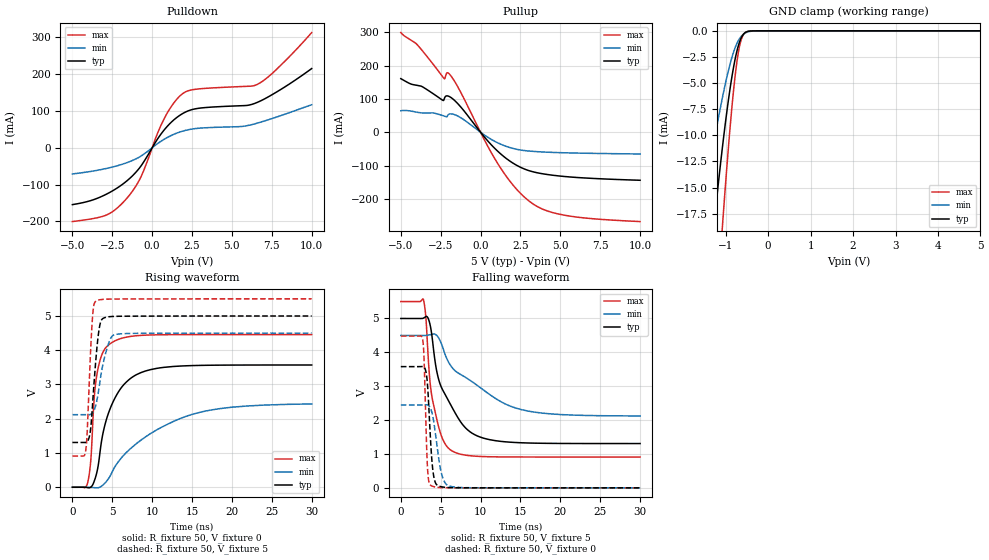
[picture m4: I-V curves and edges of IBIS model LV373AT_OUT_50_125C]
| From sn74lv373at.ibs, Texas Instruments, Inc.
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[Model]   LV373AT_OUT_50_125C
Model_type  3-state
Enable   Active-Low
Vref =   0
Rref =   1000
Cref =   50p
Vmeas =   1.5
| variable   typ   min   max
C_comp   4.53pF   3.43pF   5.27pF
| C_pullup   7.19pF   3.83pF   11.86pF
| C_pulldown   6.90pF   4.00pF   11.55pF
| C_tri-state   4.53pF   3.43pF   5.27pF
[Temperature Range]   40   140   -40
| Ambient temperature   25   125   -40
[Voltage range]   5   4.5   5.5
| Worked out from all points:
|   slope of the pulldown table from 0 to 0.75 V, typ, clamps not added: 15.5 ohm
|   slope of the pullup table from 0 to 0.75 V, typ, clamps not added: 18 ohm
|   GND clamp passes 1 mA (typ) near -0.67 V on its own axis
|   rising waveform, R_fixture 50, V_fixture 0: 20-80 % time 2.69ns typ, 7.84ns min, 968ps max; typ from 0 V to 3.57 V
|   falling waveform, R_fixture 50, V_fixture 5: 20-80 % time 3.21ns typ, 6.74ns min, 1.45ns max; typ from 5 V to 1.31 V
|   rising waveform, R_fixture 50, V_fixture 5: 20-80 % time 740ps typ, 1.19ns min, 517ps max; typ from 1.31 V to 5 V
|   falling waveform, R_fixture 50, V_fixture 0: 20-80 % time 533ps typ, 912ps min, 336ps max; typ from 3.58 V to 0 V
[GND Clamp]
| LV373AT_OUT_50
|   Voltage   I(typ)   I(min)   I(max)
-5V       -241.3mA   -136.9mA   -307.6mA
-1.61V    -33.25mA   -18.89mA   -52.32mA
-1.56V    -30.91mA   -17.58mA   -48.95mA
-1.28V    -18.74mA   -10.73mA   -30.78mA
-1.08V    -11.23mA   -6.435mA   -18.84mA
-1.06V    -10.54mA   -6.041mA   -17.72mA
-885mV    -5.19mA    -2.991mA   -8.691mA
-760mV    -2.35mA    -1.429mA   -3.693mA
-705mV    -1.458mA   -953uA     -2.131mA
-645mV    -761.3uA   -579.1uA   -987.1uA
-510mV    -98.14uA   -154.9uA   -87.32uA
5V        79.3nA     27.9nA     758.3nA
[Pulldown]
| LV373AT_OUT_50
|   Voltage   I(typ)   I(min)   I(max)
-5V       -154.5mA   -71.11mA   -200.6mA
-2.855V   -125.8mA   -56.09mA   -182.5mA
-1.595V   -90.3mA    -40.62mA   -137.6mA
-700mV    -49.38mA   -22.51mA   -78.76mA
325mV     23.07mA    10.91mA    38.05mA
815mV     51.71mA    24.74mA    84.22mA
1.34V     75.09mA    36.26mA    120.9mA
1.87V     91.96mA    44.71mA    145.8mA
2.85V     107mA      52.82mA    159.7mA
6.575V    123.1mA    66.81mA    172mA
7.735V    149.9mA    82.58mA    210.6mA
10V       215.3mA    116.9mA    313.1mA
[Pullup]
| LV373AT_OUT_50
|   Voltage   I(typ)   I(min)   I(max)
-5V       160.9mA    64.52mA    299.3mA
-3.98V    140.8mA    60.08mA    263.3mA
-2.285V   99.16mA    48.6mA     161.1mA
-2.09V    109.1mA    47.77mA    178.5mA
-1.855V   104.2mA    55.17mA    169mA
-1.215V   74.38mA    42.82mA    117.4mA
1.08V     -57.26mA   -31.9mA    -94.33mA
2.055V    -93.47mA   -48.93mA   -159.9mA
3.015V    -115mA     -56.42mA   -205.7mA
3.945V    -125.2mA   -59.41mA   -232.1mA
5.19V     -132.6mA   -61.66mA   -248.6mA
10V       -144.3mA   -65.34mA   -268.3mA
[Ramp]
| LV373AT_OUT_50
| variable   typ   min   max
dV/dt_r   2.15/2.69E-09   1.47/7.83E-09   2.75/5.21E-10
dV/dt_f   2.25/3.20E-09   1.45/6.72E-09   2.80/1.45E-09
R_load = 50
[Rising Waveform]
| LV373AT_OUT_50
R_fixture =   50
C_fixture =   0
L_fixture =   0
V_fixture =   0
V_fixture_min = 0
V_fixture_max = 0
|   Time   V(typ)   V(min)   V(max)
0s        1.266nV    7.33nV     2.497nV
1.9ns     -11mV      552.6uV    120.7mV
2.285ns   409.9uV    -2.319mV   733.8mV
2.71ns    162.6mV    -11.83mV   2.537V
3.085ns   456.2mV    -17.34mV   3.314V
3.9ns     1.651V     81.09mV    3.975V
4.94ns    2.413V     425.5mV    4.223V
8.04ns    3.288V     1.276V     4.424V
14.29ns   3.547V     2.074V     4.457V
29.99ns   3.569V     2.433V     4.457V
[Falling Waveform]
| LV373AT_OUT_50
R_fixture =   50
C_fixture =   0
L_fixture =   0
V_fixture =   5
V_fixture_min = 4.5
V_fixture_max = 5.5
|   Time   V(typ)   V(min)   V(max)
0s        5V         4.5V       5.5V
2.83ns    5.01V      4.5V       5.561V
3.145ns   5.054V     4.499V     5.024V
3.43ns    5.004V     4.507V     3.87V
3.95ns    4.398V     4.536V     2.628V
4.77ns    3.181V     4.415V     1.778V
6.34ns    2.414V     3.578V     1.102V
11.21ns   1.419V     2.745V     917.9mV
16.88ns   1.319V     2.231V     910.5mV
29.99ns   1.308V     2.121V     910.3mV
[Rising Waveform]
| LV373AT_OUT_50
R_fixture =   50
C_fixture =   0
L_fixture =   0
V_fixture =   5
V_fixture_min = 4.5
V_fixture_max = 5.5
|   Time   V(typ)   V(min)   V(max)
0s        1.308V     2.119V     910.3mV
1.665ns   1.309V     2.118V     1.067V
1.85ns    1.332V     2.117V     1.595V
2.17ns    1.527V     2.12V      3.388V
2.49ns    2.286V     2.164V     4.862V
2.98ns    3.835V     2.444V     5.438V
3.6ns     4.863V     3.309V     5.479V
4.51ns    4.976V     4.182V     5.492V
5.27ns    4.988V     4.453V     5.494V
29.99ns   5V         4.5V       5.5V
[Falling Waveform]
| LV373AT_OUT_50
R_fixture =   50
C_fixture =   0
L_fixture =   0
V_fixture =   0
V_fixture_min = 0
V_fixture_max = 0
|   Time   V(typ)   V(min)   V(max)
0s        3.579V     2.446V     4.481V
2.735ns   3.583V     2.447V     4.389V
2.92ns    3.569V     2.448V     3.78V
3.34ns    3.063V     2.451V     616.9mV
3.75ns    1.319V     2.333V     72.66mV
4.01ns    535.7mV    2.106V     44.57mV
4.325ns   159.4mV    1.628V     23.33mV
5.09ns    31.98mV    431.8mV    6.373mV
5.975ns   8.914mV    61.06mV    2.356mV
29.99ns   289.3nV    9.223uV    8.501nV
